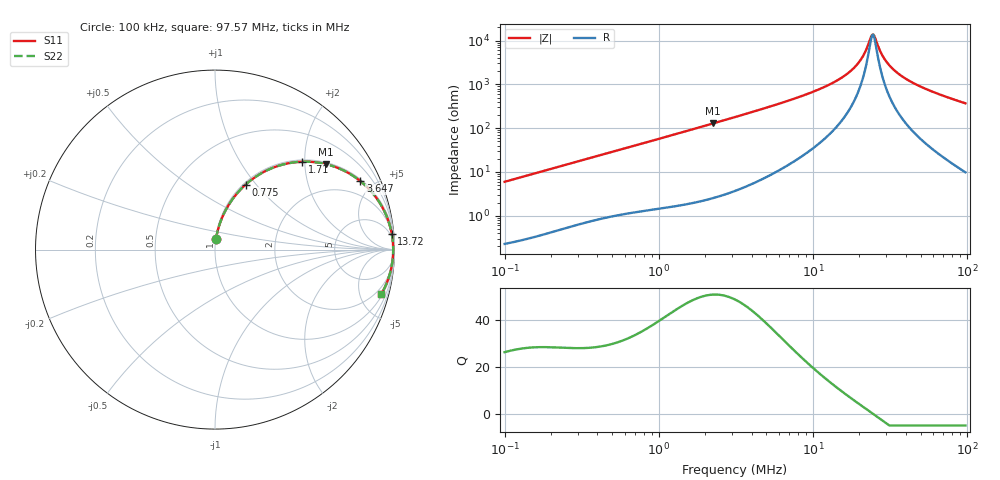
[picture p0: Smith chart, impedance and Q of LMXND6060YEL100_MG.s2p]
! LMXND6060YEL100_MG  S-PARAMETER MODEL  ( General Type )
! Model Generated by TAIYO YUDEN Corporation (https://www.yuden.co.jp/en/)
! Version 1.0
! TAIYO YUDEN Control No. 191025NI43SB-FBB
! Copyright(c) 2019 TAIYO YUDEN CO.,LTD. All Rights Reserved.
! Product Description (link to TY-COMPAS)
! https://ds.yuden.co.jp/TYCOMPAS/or/detail?pn=LMXND6060YEL100MMG&u=M
! Products Name : Inductors
! Characteristics :
!  Inductance : 10 uH , SRF(min) : 12 MHz , DC Resistance(max) : 0.0598 Ohm
!  Rated Current : Saturation :3100 mA , Temp Rise : 2400 mA (40 degC)
!  Case Size : 6.0 x 6.0 / 0.236 x 0.236 [mm/inch] , Thickness : 4.5 / 0.177 [mm/inch]
!  (Conditions: Temperature = 25 degC , DC Bias Current/Voltage = 0A / 0V)
! External Node Assignments :
!  1  o---GGG---o  2
! GND o---------o GND
! Frequency Range : 0.1MHz  -  97.572838MHz  [ 402 STEP ]
# MHz S RI R 50
! Freq[MHz].  S11 Real  S11 Imag  S21 Real  S21 Imag  S12 Real  S12 Imag  S22 Real  S22 Imag
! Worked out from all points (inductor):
!   401 points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, 100 kHz to 97.57 MHz, reference 50 ohm
!   read as one part in series: L = 9.43 uH near 103.5 kHz
!   highest Q = 50.7 at 2.253 MHz (marker M1), where L = 9.05 uH
!   self-resonance near 24.21 MHz
!   S11 on the Smith chart (normalised r, x): 100 kHz: 1.00, +0.12; 775 kHz: 1.03, +0.88; 1.71 MHz: 1.04, +1.94; 3.647 MHz: 1.09, +4.20; 13.72 MHz: 3, +22; 97.57 MHz: 1.20, -7.39
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0.1  0.00576 0.059  0.9942 -0.059  0.9942 -0.059  0.00576 0.059
0.316747  0.0388 0.1761  0.9612 -0.1761  0.9612 -0.1761  0.0388 0.1761
0.775042  0.1703 0.3619  0.8297 -0.3619  0.8297 -0.3619  0.1703 0.3619
1.003287  0.2507 0.421  0.7493 -0.421  0.7493 -0.421  0.2507 0.421
1.710402  0.4854 0.4896  0.5146 -0.4896  0.5146 -0.4896  0.4854 0.4896
2.252534  0.6192 0.4758  0.3808 -0.4758  0.3808 -0.4758  0.6192 0.4758
3.177882  0.7638 0.4145  0.2362 -0.4145  0.2362 -0.4145  0.7638 0.4145
3.646904  0.8101 0.3815  0.1899 -0.3815  0.1899 -0.3815  0.8101 0.3815
5.704673  0.9138 0.2667  0.0862 -0.2667  0.0862 -0.2667  0.9138 0.2667
9.894118  0.9709 0.1447  0.0291 -0.1447  0.0291 -0.1447  0.9709 0.1447
13.72051  0.985 0.0868  0.015 -0.0868  0.015 -0.0868  0.985 0.0868
16.5797  0.9895 0.057  0.0105 -0.057  0.0105 -0.057  0.9895 0.057
19.35694  0.9916 0.0339  0.00836 -0.0339  0.00836 -0.0339  0.9916 0.0339
21.46232  0.9925 0.0189  0.00754 -0.0189  0.00754 -0.0189  0.9925 0.0189
24.20972  0.9928 0.00168  0.00716 -0.00168  0.00716 -0.00168  0.9928 0.00168
25.05743  0.9928 -0.00324  0.00717 0.00324  0.00717 0.00324  0.9928 -0.00324
28.26505  0.9924 -0.0205  0.00757 0.0205  0.00757 0.0205  0.9924 -0.0205
31.33933  0.9916 -0.0355  0.00841 0.0355  0.00841 0.0355  0.9916 -0.0355
37.22399  0.9891 -0.0613  0.0109 0.0613  0.0109 0.0613  0.9891 -0.0613
47.36411  0.9827 -0.1002  0.0173 0.1002  0.0173 0.1002  0.9827 -0.1002
65.68142  0.9662 -0.1605  0.0338 0.1605  0.0338 0.1605  0.9662 -0.1605
97.57284  0.926 -0.2488  0.074 0.2488  0.074 0.2488  0.926 -0.2488
